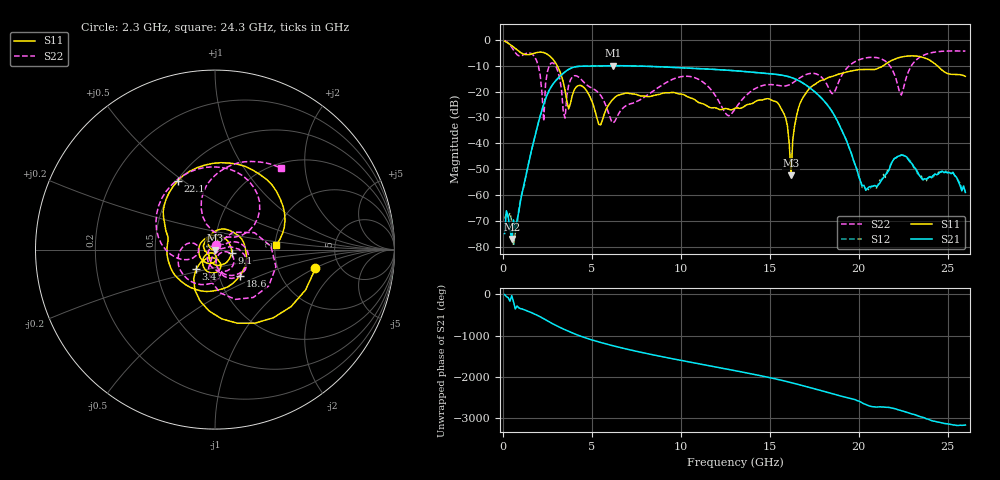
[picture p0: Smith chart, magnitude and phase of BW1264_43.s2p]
!Keysight Technologies,N5245B,MY57181159,A.13.60.06
!Date: Friday, December 18, 2020 23:54:21
!Correction: S11(Full 2 Port(1,2))
!S21(Full 2 Port(1,2))
!S12(Full 2 Port(1,2))
!S22(Full 2 Port(1,2))
!S2P File: Measurements: S11, S21, S12, S22:
# Hz S  dB  R 50
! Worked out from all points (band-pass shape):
!   260 points, 100 MHz to 26 GHz, reference 50 ohm
!   highest |S21| = -9.96 dB at 6.2 GHz (marker M1); lowest = -77.0 dB at 500 MHz (marker M2)
!   |S21| within 3 dB of the highest: 3.391 GHz to 14.84 GHz (11.45 GHz wide, 126 % of centre)
!   lowest |S11| = -52.4 dB at 16.2 GHz (marker M3), VSWR 1.00, Z = 49.8 - j0.173 ohm
!   |S11| at or under -10 dB: 3.057 GHz to 21.38 GHz (18.33 GHz wide, 150 % of centre); 24.42 GHz to end of sweep
!   |S22| runs from -32.1 to -0.2 dB; largest |S21 - S12| = 0.0006
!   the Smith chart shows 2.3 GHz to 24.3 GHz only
!   S11 on the Smith chart (normalised r, x): 2.3 GHz: 3.30, -1.02; 3.4 GHz: 0.79, -0.18; 9.1 GHz: 1.20, -0.05; 18.6 GHz: 1.26, -0.38; 22.1 GHz: 0.50, +0.48; 24.3 GHz: 2.03, +0.12
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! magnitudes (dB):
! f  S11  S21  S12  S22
! 100 MHz  -0.5  -75.0  -69.2  -0.2
! 500 MHz  -2.2  -77.0  -70.1  -2.9
! 600 MHz  -2.8  -69.7  -79.9  -3.9
! 1.9 GHz  -4.9  -34.7  -34.7  -8.1
! 2.3 GHz  -4.9  -24.9  -24.9  -31.5
! 2.7 GHz  -6.6  -18.4  -18.4  -9.1
! 3.4 GHz  -16.4  -12.9  -12.9  -28.0
! 4.5 GHz  -18.0  -10.2  -10.2  -16.0
! 6.2 GHz  -22.9  -10.0  -10.0  -32.1
! 8.8 GHz  -21.1  -10.4  -10.4  -18.1
! 9.1 GHz  -20.5  -10.5  -10.5  -16.8
! 13.1 GHz  -26.3  -12.0  -12.0  -26.3
! 15.5 GHz  -24.8  -13.4  -13.4  -17.7
! 16.2 GHz  -52.4  -14.5  -14.5  -17.0
! 16.5 GHz  -29.7  -15.3  -15.3  -15.6
! 17.4 GHz  -17.8  -19.3  -19.3  -12.9
! 18.6 GHz  -13.9  -28.8  -28.8  -20.6
! 20.2 GHz  -11.5  -56.4  -57.1  -7.3
! 21.7 GHz  -8.5  -50.5  -50.0  -9.5
! 22.1 GHz  -7.2  -45.6  -45.7  -15.1
! 24.3 GHz  -9.3  -51.9  -51.8  -4.7
! 26 GHz  -14.1  -59.1  -58.7  -4.3
